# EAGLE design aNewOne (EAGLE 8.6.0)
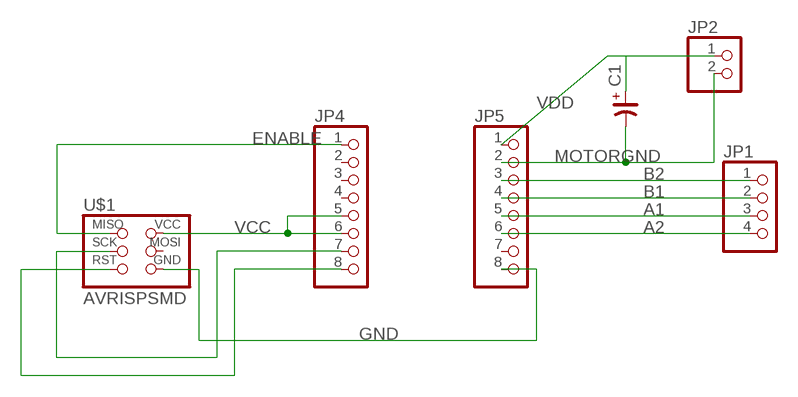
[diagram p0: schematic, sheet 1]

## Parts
C1  CP_SV-G  [CSV-G]
JP1  PINHD-1X04_2.54-SMD  [1X04SMD]
JP2  PINHD-1X02_2.54-SMD  [1X02SMD]
JP4  PINHD-1X08_2.54-SMD-90°  [1X08SMD/90]
JP5  PINHD-1X08_2.54-SMD-90°  [1X08SMD/90]
U$1  AVRISPSMD  [2X03SMD]

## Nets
A1: JP1.3 JP5.5
A2: JP1.4 JP5.6
B1: JP1.2 JP5.4
B2: JP1.1 JP5.3
ENABLE: JP4.1 U$1.1(MISO)
GND: JP5.8 U$1.6(GND)
MOTORGND: C1.- JP2.2 JP5.2
N$1: JP4.7 U$1.3(SCK)
N$2: JP4.8 U$1.5(RST)
VCC: JP4.5 JP4.6 U$1.2(VCC)
VDD: C1.+ JP2.1 JP5.1
Unconnected: JP4.2 JP4.3 JP4.4 JP5.7 U$1.4(MOSI)

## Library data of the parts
C1 = rc-master-smd:CP_: POLARIZED CAP
JP1 = pinhead-2:PINHD-1X04: PIN HEADER
JP2 = pinhead-2:PINHD-1X02: PIN HEADER
JP4 JP5 = pinhead-2:PINHD-1X08: PIN HEADER
U$1 = fab:AVRISP

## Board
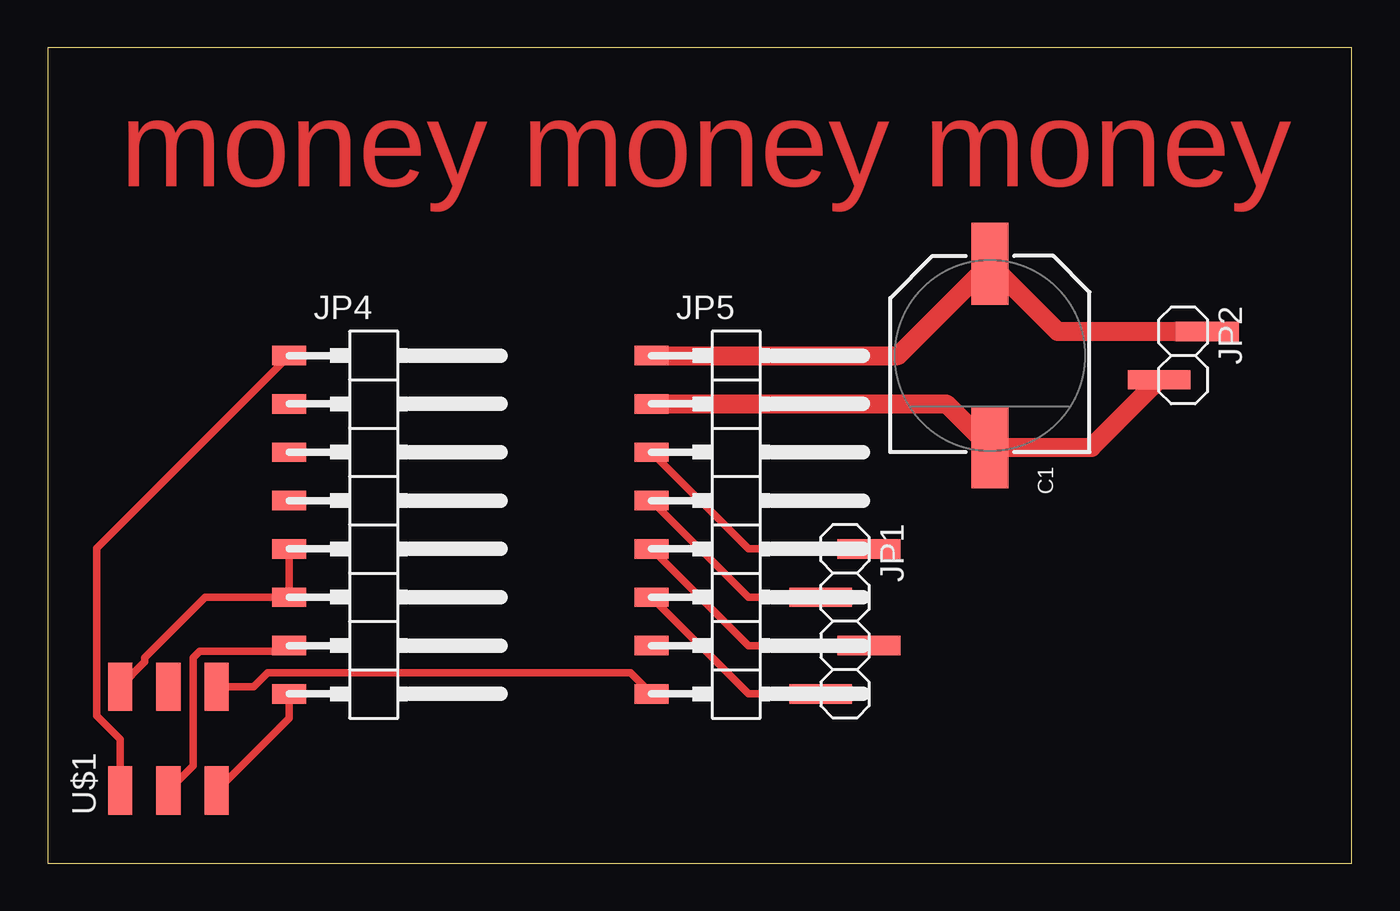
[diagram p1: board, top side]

Size 68.56 x 42.85 mm. Coordinates in mm from the lower left corner, seen from the top.
Outline: 0,0 68.56,0 68.56,42.85 0,42.85 0,0
Copper layers (1*16): Top 0.035mm / dielectric 1.5mm / Bottom 0.035mm
Design rules "default *": minimum track width 6mil, minimum drill 0.35mm, track to track 0.4mm, track to pad 0.4mm, pad to pad 0.4mm, via to via 6mil, smd to smd 6mil, copper to edge 40mil, drill to drill 6mil, minimum pad ring 10mil, minimum via ring 8mil, stop-mask expansion 4mil, vias tented up to drill 0mil, thermal gap 10mil

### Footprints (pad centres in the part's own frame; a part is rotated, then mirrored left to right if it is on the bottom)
CSV-G = smd 4.318 x 1.93: + -4.826,0; - 4.826,0
1X04SMD = smd 1.016 x 3.302: 1 -1.27,1.27; 2 1.27,-1.27; 3 3.81,1.27; 4 6.35,-1.27
1X02SMD = smd 1.016 x 3.302: 1 -1.27,1.27; 2 1.27,-1.27
1X08SMD/90 = smd 1.016 x 1.778: 1 -1.27,-5.08; 2 1.27,-5.08; 3 3.81,-5.08; 4 6.35,-5.08; 5 8.89,-5.08; 6 11.43,-5.08; 7 13.97,-5.08; 8 16.51,-5.08
2X03SMD = smd 2.54 x 1.27: 1 -2.54,2.54; 2 2.92,2.54; 3 -2.54,0; 4 2.92,0; 5 -2.54,-2.54; 6 2.92,-2.54

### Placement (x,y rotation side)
C1  49.53,26.67 270 top
JP1  41.91,15.24 270 top
JP2  59.69,26.67 270 top
JP4  17.78,25.4 270 top
JP5  36.83,25.4 270 top
U$1  6.35,6.35 90 top

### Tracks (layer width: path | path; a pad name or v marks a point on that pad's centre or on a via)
A1
  Top 0.4: JP5.5 36.83,11.43 JP1.3
A2
  Top 0.4: JP5.6 36.83,8.89 JP1.4
B1
  Top 0.4: JP5.4 36.83,13.97 JP1.2
B2
  Top 0.4: JP5.3 36.83,16.51 JP1.1
ENABLE
  Top 0.4: U$1.1 3.81,6.52 2.58,7.75 2.58,16.55 JP4.1
GND
  Top 0.4: U$1.6 10.83,9.27 11.56,10 30.64,10 JP5.8
MOTORGND
  Top 1: JP5.2 47.24,24.13 C1.- 54.86,21.84 JP2.2
N$1
  Top 0.4: U$1.3 7.66,5.12 7.66,10.79 8.01,11.14 12.41,11.14 JP4.7
N$2
  Top 0.4: U$1.5 12.7,7.62 JP4.8
VCC
  Top 0.4: JP4.5 JP4.6 8.3,13.97 5.12,10.79 5.12,10.57 U$1.2
VDD
  Top 1: JP5.1 44.7,26.67 C1.+ 53.09,27.94 JP2.1

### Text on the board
Top: money money money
